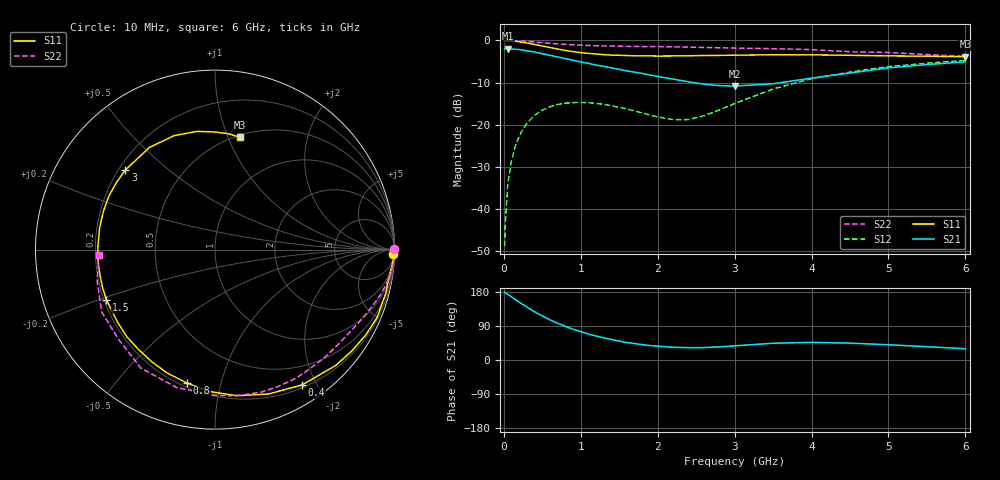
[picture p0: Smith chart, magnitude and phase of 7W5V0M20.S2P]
! Infineon Technologies  Discrete & RF Semiconductors
! BFS17W
! Si NPN RF Bipolar Junction Transistor in SOT323
! VCE = 5 V  IC = 0.2 mA
! Common Emitter S-Parameters:  August  1999
# GHz  S  MA  R  50
!  f  S11  S21  S12  S22
! GHz  MAG  ANG  MAG  ANG  MAG  ANG  MAG  ANG
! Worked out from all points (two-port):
!   36 points, 10 MHz to 6 GHz, reference 50 ohm
!   highest |S21| = -1.95 dB at 50 MHz (marker M1); lowest = -10.8 dB at 3 GHz (marker M2)
!   |S21| within 3 dB of the highest: start of sweep to 958.5 MHz
!   lowest |S11| = -3.9 dB at 6 GHz (marker M3), VSWR 4.57, Z = 25.9 + j55 ohm
!   |S11| at or under -10 dB: nowhere
!   |S22| runs from -3.8 to 0.0 dB; largest |S21 - S12| = 0.8
!   S11 on the Smith chart (normalised r, x): 10 MHz: 34, -72; 400 MHz: 0.24, -1.81; 800 MHz: 0.22, -0.79; 1.5 GHz: 0.21, -0.21; 3 GHz: 0.23, +0.36; 6 GHz: 0.52, +1.10
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0.01  0.9895 -1.3  0.797 179.4  0.0036 82.5  0.9999 0.1
0.02  0.9956 -3.2  0.797 177.4  0.0069 91.4  0.9846 -0.7
0.05  0.9843 -7.4  0.799 173.1  0.0193 86.6  0.9982 -2.1
0.1  0.9819 -14.7  0.788 166.5  0.0375 81.0  0.9955 -4.1
0.15  0.9789 -22.8  0.786 159.4  0.0559 75.5  0.9914 -6.1
0.25  0.9481 -36.7  0.768 146.0  0.0887 66.8  0.9791 -9.8
0.4  0.8967 -57.2  0.729 127.2  0.1293 55.0  0.9562 -15.1
0.6  0.8234 -81.5  0.665 106.0  0.163 41.7  0.9242 -21.1
0.8  0.7602 -101.8  0.608 88.9  0.1799 31.7  0.8986 -26.7
1.1  0.7002 -127.9  0.534 68.6  0.1824 20.8  0.8724 -34.5
1.5  0.6666 -155.2  0.454 49.8  0.1603 14.2  0.8562 -45.2
1.9  0.6551 -176.7  0.388 38.2  0.1298 17.9  0.8462 -56.7
2.2  0.6544 169.4  0.347 33.6  0.1148 30.9  0.8395 -65.5
2.4  0.6575 161.0  0.323 32.5  0.1149 43.1  0.8347 -71.8
2.6  0.6625 153.1  0.302 32.7  0.1274 54.6  0.8258 -77.9
3  0.668 138.4  0.287 37.4  0.1779 67.1  0.8118 -89.8
3.5  0.6764 122.7  0.306 44.2  0.2649 68.3  0.798 -105.4
4  0.6747 109.7  0.357 46.5  0.3517 62.4  0.7788 -122.0
4.5  0.6662 98.6  0.411 44.5  0.4214 54.7  0.7334 -137.5
5  0.6554 90.3  0.473 40.2  0.489 47.2  0.7203 -151.1
5.5  0.6499 83.1  0.517 35.1  0.5369 39.8  0.6797 -165.1
6  0.6409 77.7  0.558 29.8  0.5788 33.1  0.6471 -177.2
